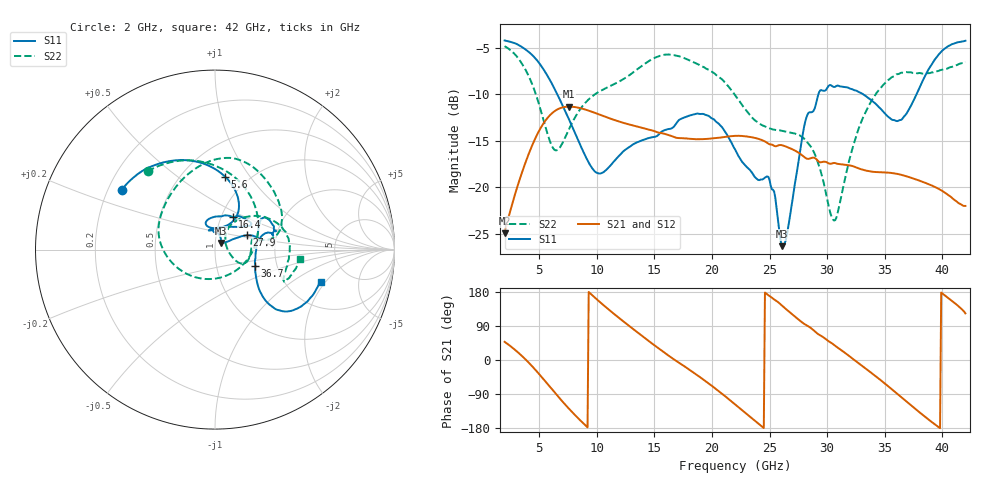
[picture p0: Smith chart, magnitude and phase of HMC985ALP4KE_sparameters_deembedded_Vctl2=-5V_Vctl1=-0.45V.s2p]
!s2p File: Measurements: S11, S21, S12, S22
# GHz S dB R 50.0
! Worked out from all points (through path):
!   401 points, 2 GHz to 42 GHz, reference 50 ohm
!   highest |S21| = -11.30 dB at 7.6 GHz (marker M1); lowest = -24.9 dB at 2 GHz (marker M2)
!   lowest |S11| = -26.3 dB at 26.1 GHz (marker M3), VSWR 1.10, Z = 53.1 + j3.9 ohm
!   |S11| at or under -10 dB: 6.581 GHz to 29.24 GHz (22.66 GHz wide, 127 % of centre); 33.16 GHz to 37.75 GHz (4.594 GHz wide, 13 % of centre)
!   |S22| runs from -23.6 to -4.8 dB; largest |S21 - S12| = 0.00028
!   S11 on the Smith chart (normalised r, x): 2 GHz: 0.26, +0.28; 5.6 GHz: 0.79, +0.77; 16.4 GHz: 1.13, +0.43; 27.9 GHz: 1.41, +0.24; 36.7 GHz: 1.54, -0.30; 42 GHz: 3.07, -1.79
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2  -4.18 147.3  -24.93 48.0  -24.93 48.0  -4.80 130.8
3.6  -4.97 120.6  -18.07 7.9  -18.07 7.9  -6.88 85.5
5.6  -7.74 82.2  -12.72 -58.7  -12.72 -58.7  -13.71 -4.6
6.5  -9.80 67.3  -11.67 -91.3  -11.67 -91.2  -16.01 -72.8
7.6  -12.70 57.4  -11.30 -129.0  -11.31 -129.0  -13.70 -138.8
8.7  -15.80 60.8  -11.51 -163.2  -11.52 -163.2  -11.35 -172.2
10.1  -18.47 86.5  -12.10 157.5  -12.10 157.5  -9.77 165.0
11.9  -16.65 109.8  -12.89 111.8  -12.90 111.8  -8.64 140.6
15.4  -14.29 76.9  -14.12 30.1  -14.12 30.1  -5.88 86.9
16.4  -13.69 61.7  -14.43 7.9  -14.44 7.9  -5.71 74.8
19.4  -12.18 34.9  -14.79 -54.8  -14.79 -54.8  -7.14 35.5
22  -15.90 52.4  -14.45 -116.9  -14.46 -116.9  -10.05 10.7
24.9  -18.88 101.7  -15.29 170.8  -15.30 170.9  -13.60 12.7
26.1  -26.32 49.3  -15.46 143.0  -15.47 143.0  -13.92 -0.5
27.9  -14.14 24.1  -16.62 97.6  -16.62 97.6  -14.63 -23.4
28.7  -11.89 12.0  -16.81 81.6  -16.81 81.6  -15.83 -28.3
30.7  -9.17 19.9  -17.39 37.4  -17.39 37.4  -23.52 23.9
32.9  -9.82 33.2  -18.03 -12.5  -18.03 -12.5  -13.13 51.1
35.4  -12.48 10.8  -18.42 -71.9  -18.43 -71.9  -8.36 21.4
36.7  -12.33 -22.1  -18.74 -104.9  -18.75 -104.9  -7.64 5.1
39.6  -5.84 -42.3  -20.10 -175.4  -20.10 -175.4  -7.49 -24.7
42  -4.22 -17.1  -21.99 122.9  -22.00 122.9  -6.48 -6.2
